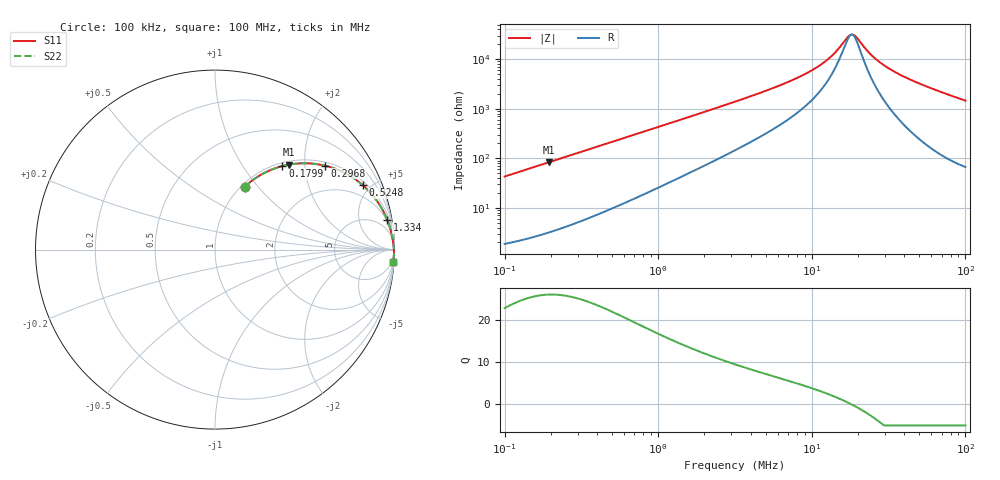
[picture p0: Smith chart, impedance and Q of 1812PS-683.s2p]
# MHz S MA R 50
!Freq  MagS11  AngS11  MagS21  AngS21  MagS12  AngS12  MagS22  AngS22
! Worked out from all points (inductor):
!   801 points, 100 kHz to 100 MHz, reference 50 ohm
!   read as one part in series: L = 68 uH near 103.5 kHz
!   highest Q = 26.1 at 194.4 kHz (marker M1), where L = 68 uH
!   self-resonance near 18.09 MHz
!   S11 on the Smith chart (normalised r, x): 100 kHz: 1.04, +0.85; 179.9 kHz: 1.06, +1.54; 296.8 kHz: 1.10, +2.53; 524.8 kHz: 1.21, +4.48; 1.334 MHz: 2, +11; 100 MHz: 2, -29
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0.1  0.3871 64.7  0.9053 -22.7  0.9053 -22.7  0.3871 64.7
0.1318257  0.4827 58.9  0.8566 -28.8  0.8566 -28.8  0.4827 58.9
0.1798871  0.5985 51.1  0.7785 -36.7  0.7785 -36.7  0.5985 51.1
0.1944241  0.6274 49.0  0.7551 -38.8  0.7551 -38.8  0.6274 49.0
0.2968247  0.7706 37.4  0.6076 -50.4  0.6076 -50.4  0.7706 37.4
0.3180534  0.7904 35.5  0.5816 -52.2  0.5816 -52.2  0.7904 35.5
0.5248075  0.8981 23.6  0.4004 -63.8  0.4004 -63.8  0.8981 23.6
1.002882  0.9613 12.9  0.224 -73.7  0.224 -73.7  0.9613 12.9
1.333521  0.9739 9.8  0.1704 -76.3  0.1704 -76.3  0.9739 9.8
3.162278  0.99 4.1  0.07143 -79.9  0.07143 -79.9  0.99 4.1
6.419482  0.9943 1.8  0.03214 -78.8  0.03214 -78.8  0.9943 1.8
10.05773  0.9957 0.9  0.0166 -74.4  0.0166 -74.4  0.9957 0.9
13.14468  0.9963 0.5  0.00921 -65.9  0.00921 -65.9  0.9963 0.5
14.70618  0.9965 0.3  0.006477 -57.0  0.006477 -57.0  0.9965 0.3
17.17908  0.9967 0.1  0.003547 -23.6  0.003547 -23.6  0.9967 0.1
18.24946  0.9968 -0.0  0.003164 2.4  0.003164 2.4  0.9968 -0.0
19.55465  0.9969 -0.1  0.003611 31.8  0.003611 31.8  0.9969 -0.1
22.64644  0.9971 -0.3  0.006408 63.0  0.006408 63.0  0.9971 -0.3
25.3367  0.9972 -0.5  0.009148 72.0  0.009148 72.0  0.9972 -0.5
31.71393  0.9974 -0.9  0.01531 79.6  0.01531 79.6  0.9974 -0.9
50.11872  0.9972 -1.8  0.03091 83.9  0.03091 83.9  0.9972 -1.8
100  0.9945 -3.9  0.06831 83.5  0.06831 83.5  0.9945 -3.9
